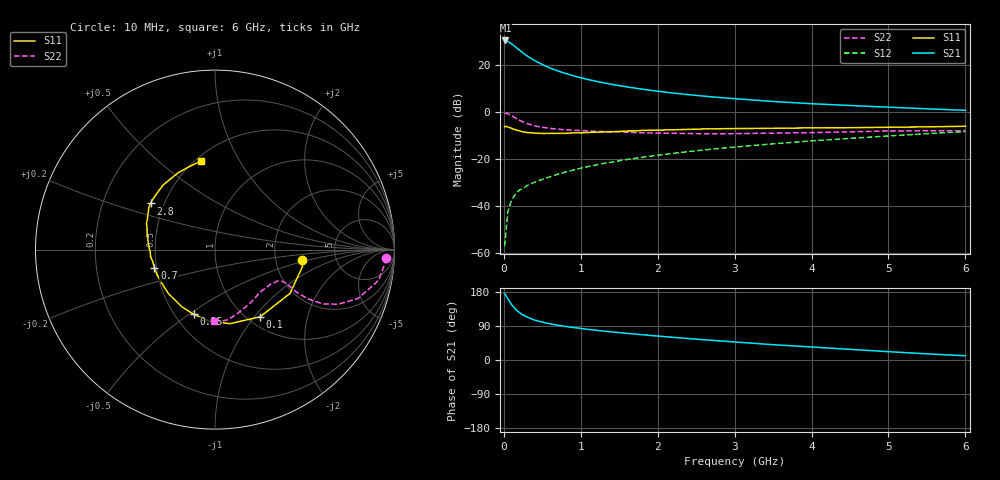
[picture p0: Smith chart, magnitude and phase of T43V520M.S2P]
! Infineon Technologies  Discrete & RF Semiconductors
! BFR182T
! Si NPN RF Bipolar Junction Transistor in SC75
! VCE = 3.5 V  IC = 20 mA
! Common Emitter S-Parameters:  October  1999
# GHz  S  MA  R  50
!  f  S11  S21  S12  S22
! GHz  MAG  ANG  MAG  ANG  MAG  ANG  MAG  ANG
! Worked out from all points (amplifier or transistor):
!   36 points, 10 MHz to 6 GHz, reference 50 ohm
!   highest |S21| = 30.5 dB at 20 MHz (marker M1)
!   |S21| within 3 dB of that: start of sweep to 160.4 MHz
!   unconditionally stable (mu >= 1): 639.3 MHz to 3.663 GHz
!   at 250 MHz: K = 0.66, MSG = 28.8 dB, |S12| = -32.5 dB
!   at 1.4 GHz: K = 1.12, MAG = 14.5 dB, |S12| = -21.4 dB
!   at 6 GHz: K = 0.84, MSG = 4.5 dB, |S12| = -8.3 dB
!   S11 on the Smith chart (normalised r, x): 10 MHz: 2.84, -0.45; 100 MHz: 1.14, -1.07; 250 MHz: 0.62, -0.52; 700 MHz: 0.49, -0.12; 2.8 GHz: 0.42, +0.27; 6 GHz: 0.53, +0.70
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0.01  0.4896 -7.1  33.43 175.0  0.0014 81.6  0.9526 -2.8
0.02  0.4966 -11.0  33.44 172.5  0.002 105.0  0.9516 -4.3
0.05  0.4839 -30.3  32.1 161.7  0.0073 84.3  0.9269 -10.7
0.1  0.4509 -56.2  28.4 146.5  0.0134 73.1  0.8421 -18.9
0.15  0.421 -78.6  24.44 134.4  0.0179 65.7  0.7509 -23.9
0.2  0.3988 -95.4  20.98 125.5  0.0218 65.5  0.6763 -26.6
0.25  0.3788 -108.4  18.08 118.7  0.0238 62.4  0.615 -27.6
0.3  0.3686 -119.7  15.78 113.4  0.0272 63.3  0.5722 -27.9
0.4  0.3571 -136.3  12.49 105.4  0.0322 62.9  0.509 -27.5
0.5  0.3508 -147.5  10.28 100.0  0.037 66.3  0.4746 -26.4
0.6  0.3518 -156.0  8.678 95.5  0.0421 66.3  0.4506 -25.8
0.7  0.3527 -162.9  7.538 91.9  0.0476 68.4  0.4332 -25.3
0.9  0.3612 -173.9  5.935 85.9  0.0581 70.1  0.4097 -25.3
1.1  0.3683 177.9  4.913 80.7  0.0697 70.9  0.3971 -26.1
1.3  0.3785 171.2  4.193 76.3  0.0809 71.3  0.3852 -27.5
1.6  0.3949 163.7  3.432 70.3  0.098 71.4  0.3718 -30.0
2.2  0.4204 153.0  2.546 59.8  0.1322 70.6  0.3542 -37.4
2.8  0.4418 144.4  2.046 50.5  0.1681 68.7  0.3449 -45.8
3.5  0.4517 134.9  1.681 40.4  0.2109 65.8  0.3565 -56.2
4.5  0.4649 122.5  1.38 28.1  0.276 60.5  0.3797 -71.8
5.5  0.4847 106.8  1.173 16.2  0.3469 54.4  0.4006 -85.2
6  0.4994 99.1  1.09 11.2  0.3843 50.5  0.4001 -90.7
